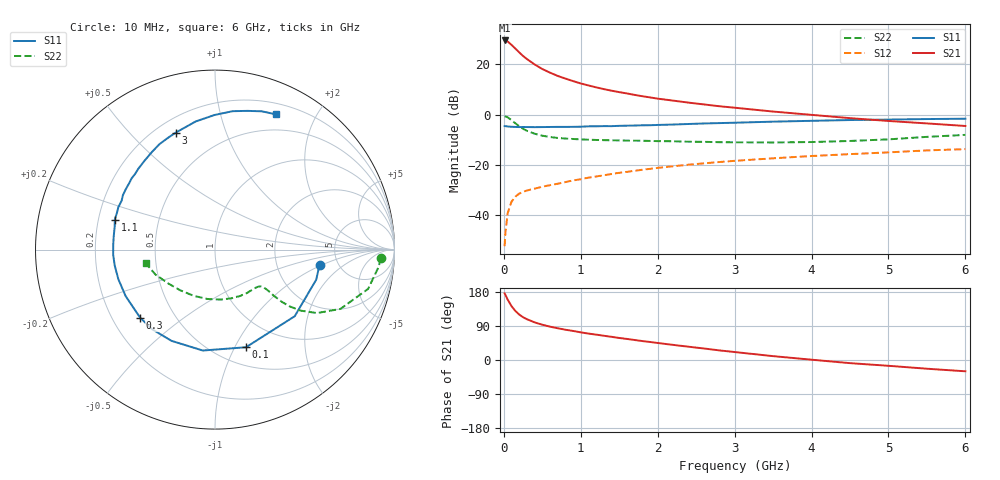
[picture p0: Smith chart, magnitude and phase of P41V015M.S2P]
! SIEMENS Small Signal Semiconductors
! BFP182
! Si NPN RF Bipolar Junction Transistor in SOT143
! VCE = 1 V  IC = 15 mA
! Common Emitter S-Parameters:  March  1996
# GHz  S  MA  R  50
!  f  S11  S21  S12  S22
! GHz  MAG  ANG  MAG  ANG  MAG  ANG  MAG  ANG
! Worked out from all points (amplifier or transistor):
!   36 points, 10 MHz to 6 GHz, reference 50 ohm
!   highest |S21| = 29.5 dB at 10 MHz (marker M1)
!   |S21| within 3 dB of that: start of sweep to 141.8 MHz
!   unconditionally stable (mu >= 1): 554.2 MHz to end of sweep
!   at 250 MHz: K = 0.56, MSG = 27.1 dB, |S12| = -30.8 dB
!   at 1.4 GHz: K = 1.44, MAG = 12.7 dB, |S12| = -23.7 dB
!   at 6 GHz: K = 1.14, MAG = 2.3 dB, |S12| = -13.8 dB
!   S11 on the Smith chart (normalised r, x): 10 MHz: 3.59, -0.95; 100 MHz: 0.69, -1.11; 300 MHz: 0.32, -0.35; 1.1 GHz: 0.27, +0.14; 3 GHz: 0.28, +0.68; 6 GHz: 0.32, +1.50
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0.01  0.5887 -8.4  29.83 175.9  0.0024 84.0  0.9237 -2.9
0.02  0.5882 -16.6  29.79 171.8  0.0044 80.9  0.9175 -5.9
0.05  0.5788 -39.9  28.44 159.3  0.0109 75.5  0.8807 -14.4
0.1  0.5708 -72.4  24.36 142.1  0.0185 59.7  0.7731 -25.3
0.15  0.5664 -96.9  20.53 129.4  0.0232 52.3  0.6693 -31.9
0.2  0.5632 -115.5  17.27 119.9  0.0267 47.7  0.5855 -35.5
0.25  0.5653 -128.1  14.63 112.9  0.0288 44.5  0.5207 -37.3
0.3  0.5639 -137.7  12.72 107.7  0.0308 43.8  0.4743 -38.0
0.4  0.5612 -152.5  9.942 99.3  0.0334 42.8  0.4152 -38.1
0.5  0.5632 -163.0  8.048 93.1  0.0366 42.8  0.3795 -37.7
0.6  0.5657 -171.0  6.829 88.0  0.0393 44.1  0.3571 -37.7
0.7  0.5681 -177.1  5.87 83.8  0.042 45.4  0.3423 -37.8
0.8  0.5677 177.0  5.199 79.9  0.0453 46.2  0.333 -38.3
1  0.5728 167.4  4.155 73.0  0.0516 47.9  0.3203 -39.9
1.1  0.5828 163.3  3.795 69.7  0.0555 48.7  0.3158 -41.1
1.5  0.596 149.4  2.793 58.1  0.0693 48.5  0.3057 -47.2
2.2  0.6325 128.2  1.894 39.9  0.0935 45.6  0.294 -61.8
3  0.6876 108.5  1.368 21.0  0.1198 39.5  0.2803 -83.2
3.5  0.7219 98.6  1.147 10.2  0.1345 35.2  0.2783 -98.7
4.5  0.7775 82.7  0.848 -8.3  0.1631 26.5  0.298 -130.4
5.5  0.8134 71.3  0.666 -23.0  0.1934 18.0  0.3595 -157.2
6  0.8259 65.9  0.592 -29.8  0.205 12.7  0.394 -169.1
